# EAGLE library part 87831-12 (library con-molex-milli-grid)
HEADER
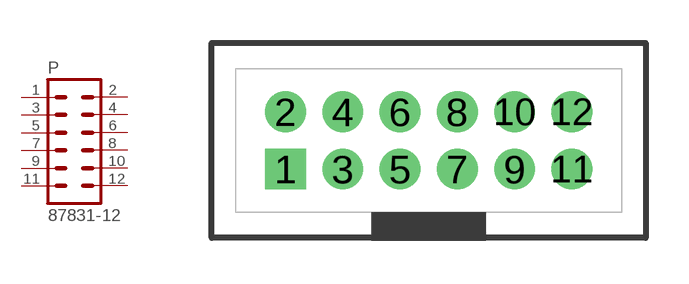
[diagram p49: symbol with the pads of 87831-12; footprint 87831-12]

Designator prefix P

## 87831-12  [87831-12]
1  1  pas
2  2  pas
3  3  pas
4  4  pas
5  5  pas
6  6  pas
7  7  pas
8  8  pas
9  9  pas
10  10  pas
11  11  pas
12  12  pas

## Footprint 87831-12 (pad centres in mm)
HEADER Dual Row, Shrouded, Vertical
drill 0.914 square: 1 -5,-1
drill 0.914: 2 -5,1; 3 -3,-1; 4 -3,1; 5 -1,-1; 6 -1,1; 7 1,-1; 8 1,1; 9 3,-1; 10 3,1; 11 5,-1; 12 5,1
